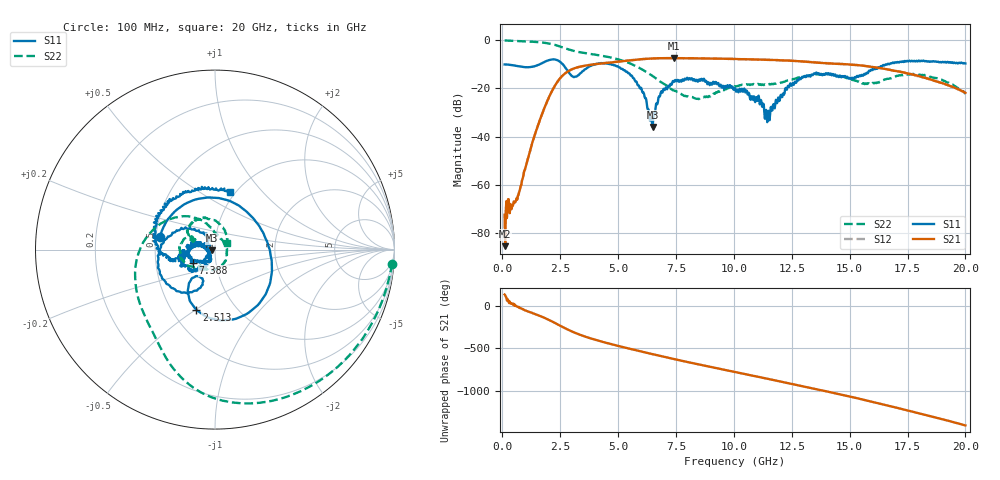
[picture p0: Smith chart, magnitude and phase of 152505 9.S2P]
!  2-Port S-parameters saved by WinCal
! VAR MeasName=S-Parameters (CALIBRATED_DATA) read from VNA (N5230C)
! VAR MeasDate=4/10/2015 9:29:15 AM
! VAR NAME=152505 9
! VAR FILENAME=152505 9.S2P
! VAR DATE=4/10/2015 9:29:15 AM
! VAR PHYS_PORTS=1,2
# Hz S DB R 50
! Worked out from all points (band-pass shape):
!   801 points, 100 MHz to 20 GHz, reference 50 ohm
!   highest |S21| = -7.41 dB at 7.413 GHz (marker M1); lowest = -85.6 dB at 124.9 MHz (marker M2)
!   |S21| within 3 dB of the highest: 3.662 GHz to 15.44 GHz (11.78 GHz wide, 123 % of centre)
!   lowest |S11| = -36.0 dB at 6.493 GHz (marker M3), VSWR 1.03, Z = 48.5 - j0.404 ohm
!   |S11| at or under -10 dB: start of sweep to 1.613 GHz; 2.616 GHz to 4.024 GHz (1.408 GHz wide, 42.4 % of centre); 4.697 GHz to 16.63 GHz (11.93 GHz wide, 112 % of centre)
!   |S22| runs from -24.5 to -0.1 dB; largest |S21 - S12| = 0.0069
!   S11 on the Smith chart (normalised r, x): 100 MHz: 0.53, +0.08; 2.513 GHz: 0.66, -0.50; 7.388 GHz: 0.77, -0.12; 20 GHz: 0.94, +0.68
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1e8  -10.05 166.8  -72.52 133.9  -81.79 39.2  -0.08 -4.6
1.24875e8  -10.06 163.5  -85.56 126.6  -80.26 59.1  -0.10 -5.5
2.4925e8  -10.11 147.0  -66.02 71.1  -66.33 78.9  -0.17 -10.5
6.72125e8  -10.78 91.9  -64.67 -12.8  -65.01 -12.3  -0.32 -27.3
1.617375e9  -9.97 -8.8  -33.24 -118.2  -33.28 -117.9  -0.84 -66.1
2.512875e9  -9.08 -107.2  -15.61 124.2  -15.61 124.3  -2.68 -105.1
3.43325e9  -13.20 -110.7  -10.84 11.6  -10.81 11.9  -5.11 -131.9
4.403375e9  -9.60 -158.1  -9.49 -69.8  -9.48 -69.8  -6.63 -162.8
5.298875e9  -12.58 153.2  -8.59 -131.4  -8.57 -131.4  -8.83 162.1
6.492875e9  -36.01 -164.7  -7.59 150.1  -7.58 150.2  -14.85 114.6
6.741625e9  -24.02 -142.4  -7.48 134.5  -7.46 134.3  -16.62 107.0
7.388375e9  -16.93 -148.9  -7.42 94.3  -7.39 94.0  -20.84 89.0
7.41325e9  -17.32 -149.1  -7.41 92.9  -7.40 92.8  -20.87 87.6
8.781375e9  -17.04 173.0  -7.56 12.6  -7.56 12.5  -23.65 -0.4
1.005e10  -19.80 166.4  -7.77 -60.0  -7.80 -60.2  -19.11 -87.3
1.1443e10  -34.04 -177.7  -8.14 -139.3  -8.13 -139.1  -18.23 -130.1
1.23385e10  -18.92 -119.3  -8.42 168.7  -8.47 168.3  -16.61 -137.6
1.338325e10  -14.42 -150.2  -9.14 107.7  -9.07 107.9  -14.30 -162.5
1.507475e10  -15.84 -173.6  -10.16 6.4  -10.12 6.8  -16.33 151.6
1.669162e10  -9.91 178.7  -12.19 -99.0  -12.23 -100.4  -16.00 156.2
1.83085e10  -8.65 129.5  -15.80 151.5  -15.71 149.8  -14.58 106.8
2e10  -9.66 75.5  -21.81 29.5  -21.86 29.8  -22.25 27.5
